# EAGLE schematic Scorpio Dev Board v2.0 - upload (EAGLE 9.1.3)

## Sheet 1 of 3: MAIN SECTION
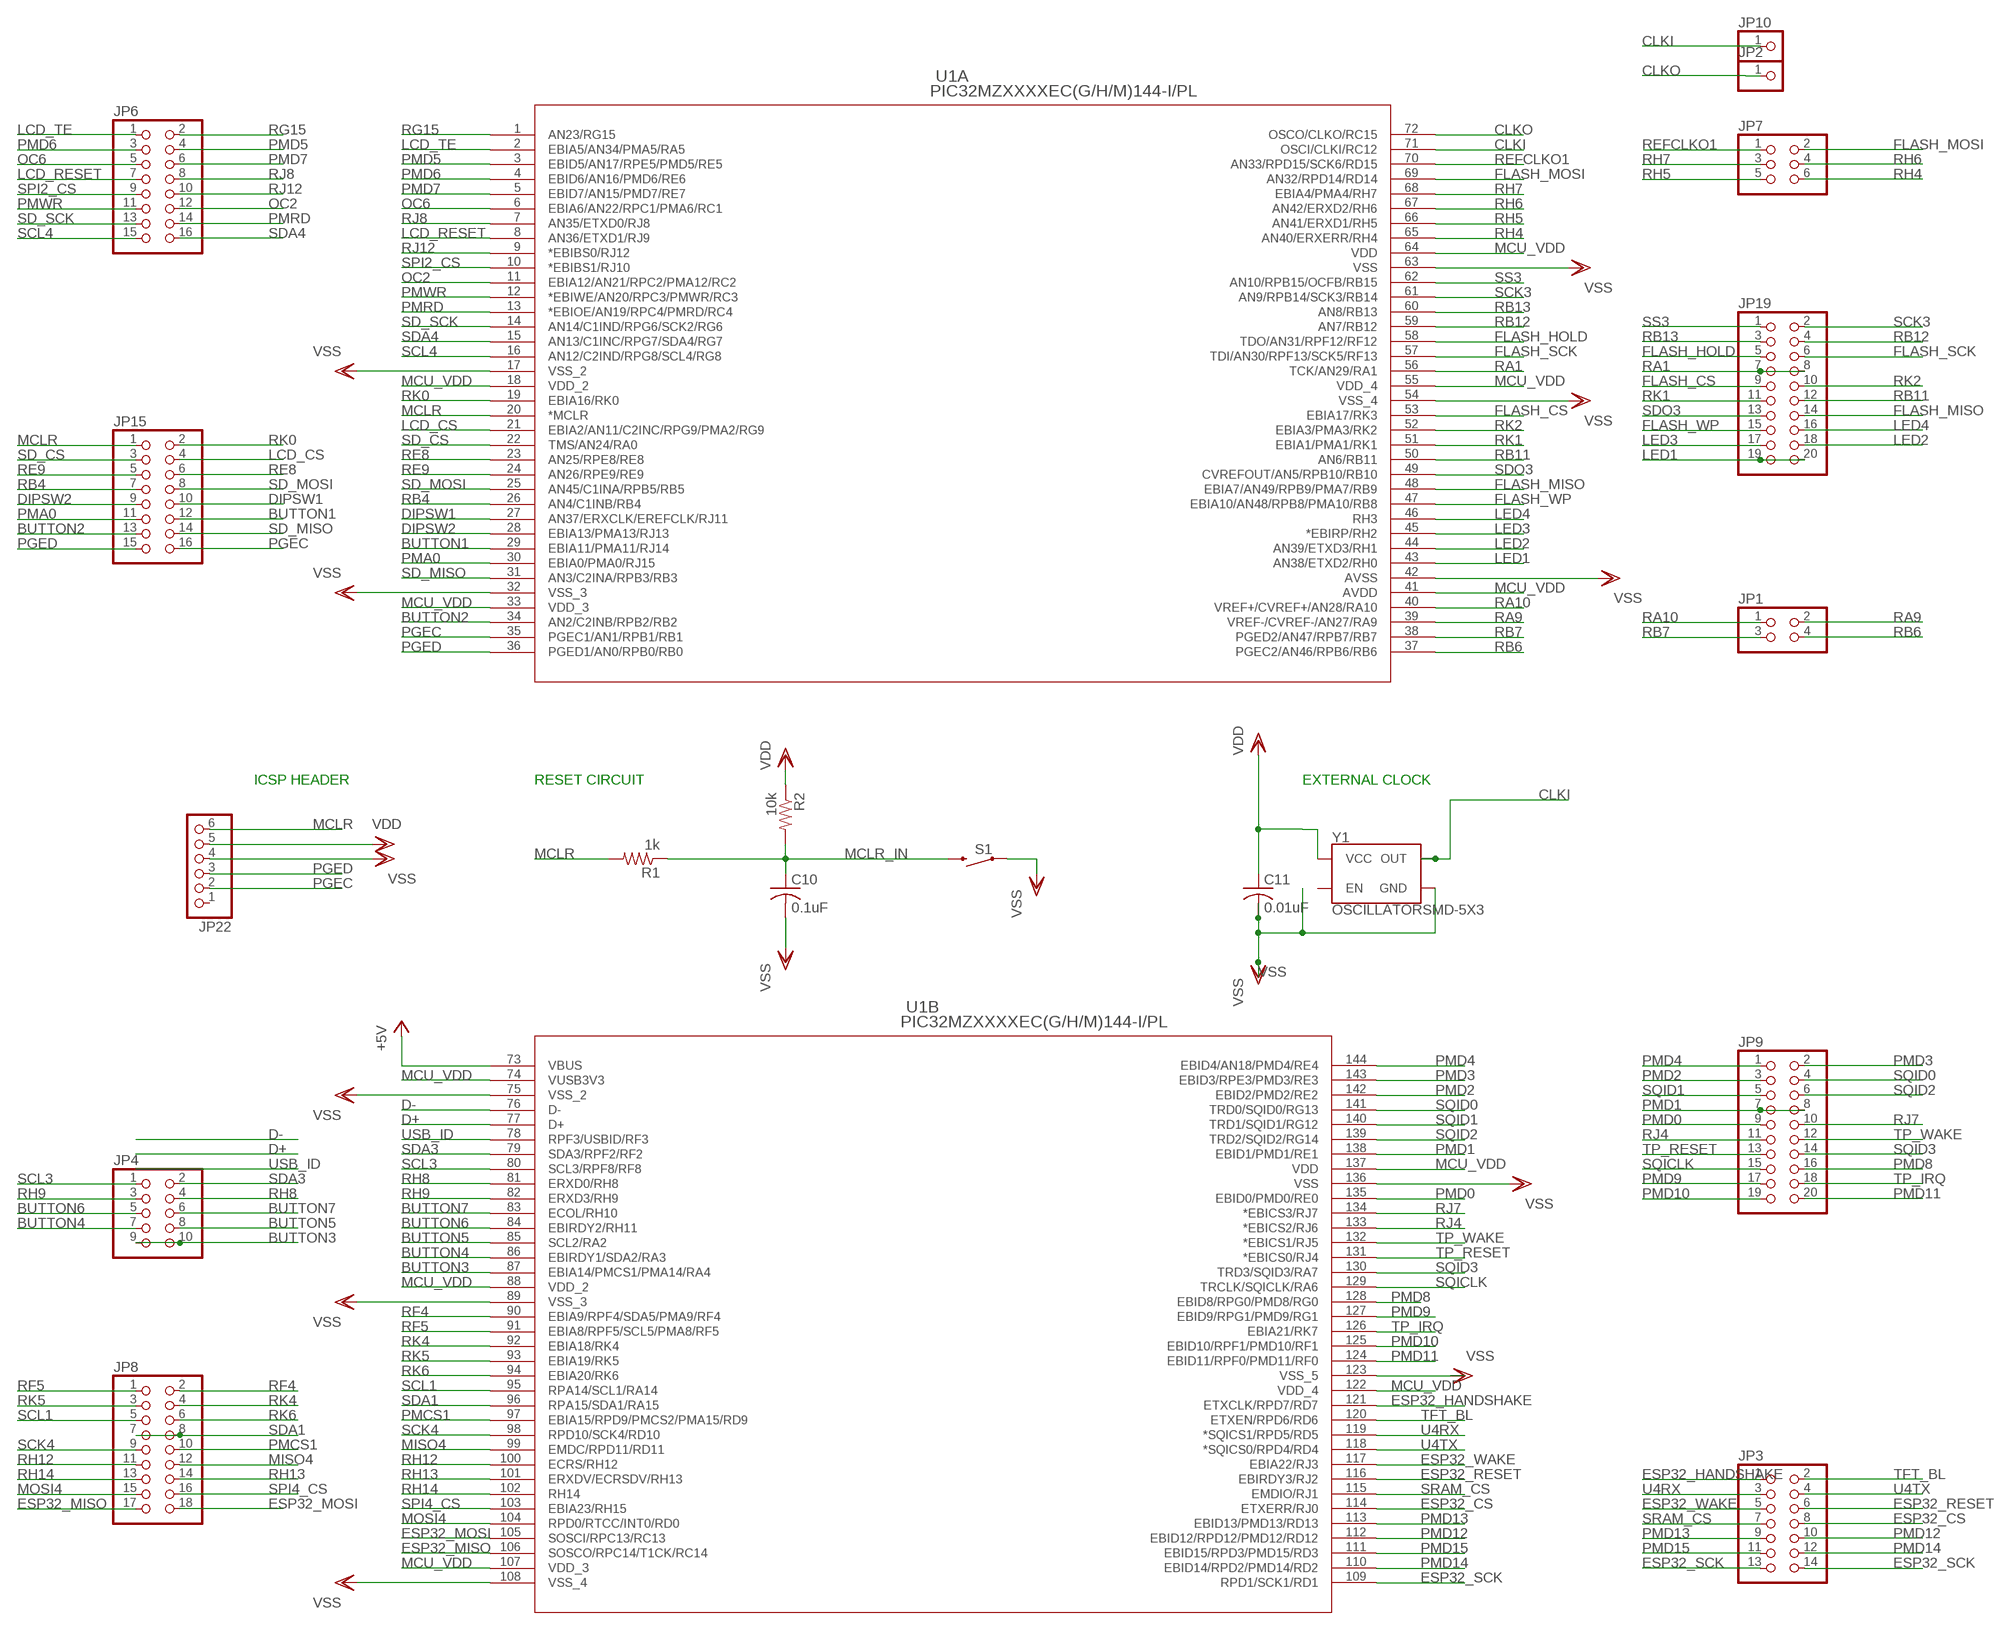
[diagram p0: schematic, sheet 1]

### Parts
C10  0.1uF  C-USC1206K  [C1206K]
C11  0.01uF  C-USC1206K  [C1206K]
JP1  PINHD-2X2  [2X02]
JP2  PINHD-1X1  [1X01]
JP3  PINHD-2X7  [2X07]
JP4  PINHD-2X5  [2X05]
JP6  PINHD-2X8  [2X08]
JP7  PINHD-2X3  [2X03]
JP8  PINHD-2X9  [2X09]
JP9  PINHD-2X10  [2X10]
JP10  PINHD-1X1  [1X01]
JP15  PINHD-2X8  [2X08]
JP19  PINHD-2X10  [2X10]
JP22  PINHD-1X6  [1X06]
R1  1k  R-US_M1206  [M1206]
R2  10k  R-US_M1206  [M1206]
S1  SWITCH-MOMENTARY-2PTH  [TACTILE-PTH]
U1  PIC32MZXXXXEC(G/H/M)144-I/PL  [LQFP144_20X20MC]
Y1  OSCILLATORSMD-5X3  [OSCILLATOR-SMD-5X3.2]

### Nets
+5V: U1.73(B:VBUS) ; also sheet 2,3
BUTTON1: JP15.12 U1.29(A:EBIA11/PMA11/RJ14) ; also sheet 2
BUTTON2: JP15.13 U1.34(A:AN2/C2INB/RPB2/RB2)
BUTTON3: JP4.9 JP4.10 U1.87(B:EBIA14/PMCS1/PMA14/RA4)
BUTTON4: JP4.7 U1.86(B:EBIRDY1/SDA2/RA3)
BUTTON5: JP4.8 U1.85(B:SCL2/RA2)
BUTTON6: JP4.5 U1.84(B:EBIRDY2/RH11)
BUTTON7: JP4.6 U1.83(B:ECOL/RH10)
CLKI: JP10.1 U1.71(A:OSCI/CLKI/RC12) Y1.3(OUT)
CLKO: JP2.1 U1.72(A:OSCO/CLKO/RC15)
D+: U1.77(B:D+) ; also sheet 2
D-: U1.76(B:D-) ; also sheet 2
DIPSW1: JP15.10 U1.27(A:AN37/ERXCLK/EREFCLK/RJ11)
DIPSW2: JP15.9 U1.28(A:EBIA13/PMA13/RJ13)
ESP32_CS: JP3.8 U1.114(B:ETXERR/RJ0) ; also sheet 2
ESP32_HANDSHAKE: JP3.1 U1.121(B:ETXCLK/RPD7/RD7) ; also sheet 2
ESP32_MISO: JP8.17 U1.106(B:SOSCO/RPC14/T1CK/RC14) ; also sheet 2
ESP32_MOSI: JP8.18 U1.105(B:SOSCI/RPC13/RC13) ; also sheet 2
ESP32_RESET: JP3.6 U1.116(B:EBIRDY3/RJ2) ; also sheet 2
ESP32_SCK: JP3.13 JP3.14 U1.109(B:RPD1/SCK1/RD1) ; also sheet 2
ESP32_WAKE: JP3.5 U1.117(B:EBIA22/RJ3) ; also sheet 2
FLASH_CS: JP19.9 U1.53(A:EBIA17/RK3) ; also sheet 2
FLASH_HOLD: JP19.5 U1.58(A:TDO/AN31/RPF12/RF12)
FLASH_MISO: JP19.14 U1.48(A:EBIA7/AN49/RPB9/PMA7/RB9) ; also sheet 2
FLASH_MOSI: JP7.2 U1.69(A:AN32/RPD14/RD14) ; also sheet 2
FLASH_SCK: JP19.6 U1.57(A:TDI/AN30/RPF13/SCK5/RF13) ; also sheet 2
FLASH_WP: JP19.15 U1.47(A:EBIA10/AN48/RPB8/PMA10/RB8) ; also sheet 2
LCD_CS: JP15.4 U1.21(A:EBIA2/AN11/C2INC/RPG9/PMA2/RG9) ; also sheet 2
LCD_RESET: JP6.7 U1.8(A:AN36/ETXD1/RJ9) ; also sheet 2
LCD_TE: JP6.1 U1.2(A:EBIA5/AN34/PMA5/RA5) ; also sheet 2
LED1: JP19.19 JP19.20 U1.43(A:AN38/ETXD2/RH0) ; also sheet 2
LED2: JP19.18 U1.44(A:AN39/ETXD3/RH1) ; also sheet 2
LED3: JP19.17 U1.45(A:*EBIRP/RH2) ; also sheet 2
LED4: JP19.16 U1.46(A:RH3) ; also sheet 2
MCLR: JP15.1 JP22.6 R1.2 U1.20(A:*MCLR)
MCLR_IN: C10.1 R1.1 R2.2 S1.3
MCU_VDD: U1.18(A:VDD_2) U1.33(A:VDD_3) U1.41(A:AVDD) U1.55(A:VDD_4) U1.64(A:VDD) U1.74(B:VUSB3V3) U1.88(B:VDD_2) U1.107(B:VDD_3) U1.122(B:VDD_4) U1.137(B:VDD) ; also sheet 2,3
MISO4: JP8.12 U1.99(B:EMDC/RPD11/RD11)
MOSI4: JP8.15 U1.104(B:RPD0/RTCC/INT0/RD0)
OC2: JP6.12 U1.11(A:EBIA12/AN21/RPC2/PMA12/RC2) ; also sheet 2
OC6: JP6.5 U1.6(A:EBIA6/AN22/RPC1/PMA6/RC1) ; also sheet 2
PGEC: JP15.16 JP22.2 U1.35(A:PGEC1/AN1/RPB1/RB1)
PGED: JP15.15 JP22.3 U1.36(A:PGED1/AN0/RPB0/RB0)
PMA0: JP15.11 U1.30(A:EBIA0/PMA0/RJ15) ; also sheet 2
PMCS1: JP8.10 U1.97(B:EBIA15/RPD9/PMCS2/PMA15/RD9)
PMD0: JP9.9 U1.135(B:EBID0/PMD0/RE0) ; also sheet 2
PMD1: JP9.7 JP9.8 U1.138(B:EBID1/PMD1/RE1) ; also sheet 2
PMD2: JP9.3 U1.142(B:EBID2/PMD2/RE2) ; also sheet 2
PMD3: JP9.2 U1.143(B:EBID3/RPE3/PMD3/RE3) ; also sheet 2
PMD4: JP9.1 U1.144(B:EBID4/AN18/PMD4/RE4) ; also sheet 2
PMD5: JP6.4 U1.3(A:EBID5/AN17/RPE5/PMD5/RE5) ; also sheet 2
PMD6: JP6.3 U1.4(A:EBID6/AN16/PMD6/RE6) ; also sheet 2
PMD7: JP6.6 U1.5(A:EBID7/AN15/PMD7/RE7) ; also sheet 2
PMD8: JP9.16 U1.128(B:EBID8/RPG0/PMD8/RG0) ; also sheet 2
PMD9: JP9.17 U1.127(B:EBID9/RPG1/PMD9/RG1) ; also sheet 2
PMD10: JP9.19 U1.125(B:EBID10/RPF1/PMD10/RF1) ; also sheet 2
PMD11: JP9.20 U1.124(B:EBID11/RPF0/PMD11/RF0) ; also sheet 2
PMD12: JP3.10 U1.112(B:EBID12/RPD12/PMD12/RD12) ; also sheet 2
PMD13: JP3.9 U1.113(B:EBID13/PMD13/RD13) ; also sheet 2
PMD14: JP3.12 U1.110(B:EBID14/RPD2/PMD14/RD2) ; also sheet 2
PMD15: JP3.11 U1.111(B:EBID15/RPD3/PMD15/RD3) ; also sheet 2
PMRD: JP6.14 U1.13(A:*EBIOE/AN19/RPC4/PMRD/RC4) ; also sheet 2
PMWR: JP6.11 U1.12(A:*EBIWE/AN20/RPC3/PMWR/RC3) ; also sheet 2
RA1: JP19.7 JP19.8 U1.56(A:TCK/AN29/RA1)
RA9: JP1.2 U1.39(A:VREF-/CVREF-/AN27/RA9)
RA10: JP1.1 U1.40(A:VREF+/CVREF+/AN28/RA10)
RB4: JP15.7 U1.26(A:AN4/C1INB/RB4)
RB6: JP1.4 U1.37(A:PGEC2/AN46/RPB6/RB6)
RB7: JP1.3 U1.38(A:PGED2/AN47/RPB7/RB7)
RB11: JP19.12 U1.50(A:AN6/RB11)
RB12: JP19.4 U1.59(A:AN7/RB12)
RB13: JP19.3 U1.60(A:AN8/RB13)
RE8: JP15.6 U1.23(A:AN25/RPE8/RE8)
RE9: JP15.5 U1.24(A:AN26/RPE9/RE9)
REFCLKO1: JP7.1 U1.70(A:AN33/RPD15/SCK6/RD15) ; also sheet 2
RF4: JP8.2 U1.90(B:EBIA9/RPF4/SDA5/PMA9/RF4)
RF5: JP8.1 U1.91(B:EBIA8/RPF5/SCL5/PMA8/RF5)
RG15: JP6.2 U1.1(A:AN23/RG15)
RH4: JP7.6 U1.65(A:AN40/ERXERR/RH4)
RH5: JP7.5 U1.66(A:AN41/ERXD1/RH5)
RH6: JP7.4 U1.67(A:AN42/ERXD2/RH6)
RH7: JP7.3 U1.68(A:EBIA4/PMA4/RH7)
RH8: JP4.4 U1.81(B:ERXD0/RH8)
RH9: JP4.3 U1.82(B:ERXD3/RH9)
RH12: JP8.11 U1.100(B:ECRS/RH12)
RH13: JP8.14 U1.101(B:ERXDV/ECRSDV/RH13)
RH14: JP8.13 U1.102(B:RH14)
RJ4: JP9.11 U1.133(B:*EBICS2/RJ6)
RJ7: JP9.10 U1.134(B:*EBICS3/RJ7)
RJ8: JP6.8 U1.7(A:AN35/ETXD0/RJ8)
RJ12: JP6.10 U1.9(A:*EBIBS0/RJ12)
RK0: JP15.2 U1.19(A:EBIA16/RK0)
RK1: JP19.11 U1.51(A:EBIA1/PMA1/RK1)
RK2: JP19.10 U1.52(A:EBIA3/PMA3/RK2)
RK4: JP8.4 U1.92(B:EBIA18/RK4)
RK5: JP8.3 U1.93(B:EBIA19/RK5)
RK6: JP8.6 U1.94(B:EBIA20/RK6)
SCK3: JP19.2 U1.61(A:AN9/RPB14/SCK3/RB14) ; also sheet 2
SCK4: JP8.9 U1.98(B:RPD10/SCK4/RD10)
SCL1: JP8.5 U1.95(B:RPA14/SCL1/RA14) ; also sheet 2
SCL3: JP4.1 U1.80(B:SCL3/RPF8/RF8)
SCL4: JP6.15 U1.16(A:AN12/C2IND/RPG8/SCL4/RG8) ; also sheet 2
SD_CS: JP15.3 U1.22(A:TMS/AN24/RA0) ; also sheet 2
SD_MISO: JP15.14 U1.31(A:AN3/C2INA/RPB3/RB3) ; also sheet 2
SD_MOSI: JP15.8 U1.25(A:AN45/C1INA/RPB5/RB5) ; also sheet 2
SD_SCK: JP6.13 U1.14(A:AN14/C1IND/RPG6/SCK2/RG6) ; also sheet 2
SDA1: JP8.7 JP8.8 U1.96(B:RPA15/SDA1/RA15) ; also sheet 2
SDA3: JP4.2 U1.79(B:SDA3/RPF2/RF2)
SDA4: JP6.16 U1.15(A:AN13/C1INC/RPG7/SDA4/RG7) ; also sheet 2
SDO3: JP19.13 U1.49(A:CVREFOUT/AN5/RPB10/RB10) ; also sheet 2
SPI2_CS: JP6.9 U1.10(A:*EBIBS1/RJ10)
SPI4_CS: JP8.16 U1.103(B:EBIA23/RH15)
SQICLK: JP9.15 U1.129(B:TRCLK/SQICLK/RA6) ; also sheet 2
SQID0: JP9.4 U1.141(B:TRD0/SQID0/RG13) ; also sheet 2
SQID1: JP9.5 U1.140(B:TRD1/SQID1/RG12) ; also sheet 2
SQID2: JP9.6 U1.139(B:TRD2/SQID2/RG14) ; also sheet 2
SQID3: JP9.14 U1.130(B:TRD3/SQID3/RA7) ; also sheet 2
SRAM_CS: JP3.7 U1.115(B:EMDIO/RJ1) ; also sheet 2
SS3: JP19.1 U1.62(A:AN10/RPB15/OCFB/RB15) ; also sheet 2
TFT_BL: JP3.2 U1.120(B:ETXEN/RPD6/RD6) ; also sheet 2
TP_IRQ: JP9.18 U1.126(B:EBIA21/RK7) ; also sheet 2
TP_RESET: JP9.13 U1.131(B:*EBICS0/RJ4) ; also sheet 2
TP_WAKE: JP9.12 U1.132(B:*EBICS1/RJ5) ; also sheet 2
U4RX: JP3.3 U1.119(B:*SQICS1/RPD5/RD5) ; also sheet 2
U4TX: JP3.4 U1.118(B:*SQICS0/RPD4/RD4) ; also sheet 2
USB_ID: U1.78(B:RPF3/USBID/RF3) ; also sheet 2
VDD: C11.1 JP22.5 R2.1 Y1.4(VCC) ; also sheet 2,3
VSS: C10.2 C11.2 JP22.4 S1.1 U1.17(A:VSS_2) U1.32(A:VSS_3) U1.42(A:AVSS) U1.54(A:VSS_4) U1.63(A:VSS) U1.75(B:VSS_2) U1.89(B:VSS_3) U1.108(B:VSS_4) U1.123(B:VSS_5) U1.136(B:VSS) Y1.2(GND) ; also sheet 2,3
Unconnected: JP22.1 Y1.1(EN)

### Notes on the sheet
- ICSP HEADER | RESET CIRCUIT | EXTERNAL CLOCK

## Sheet 2 of 3: PERIPHERALS SECTION
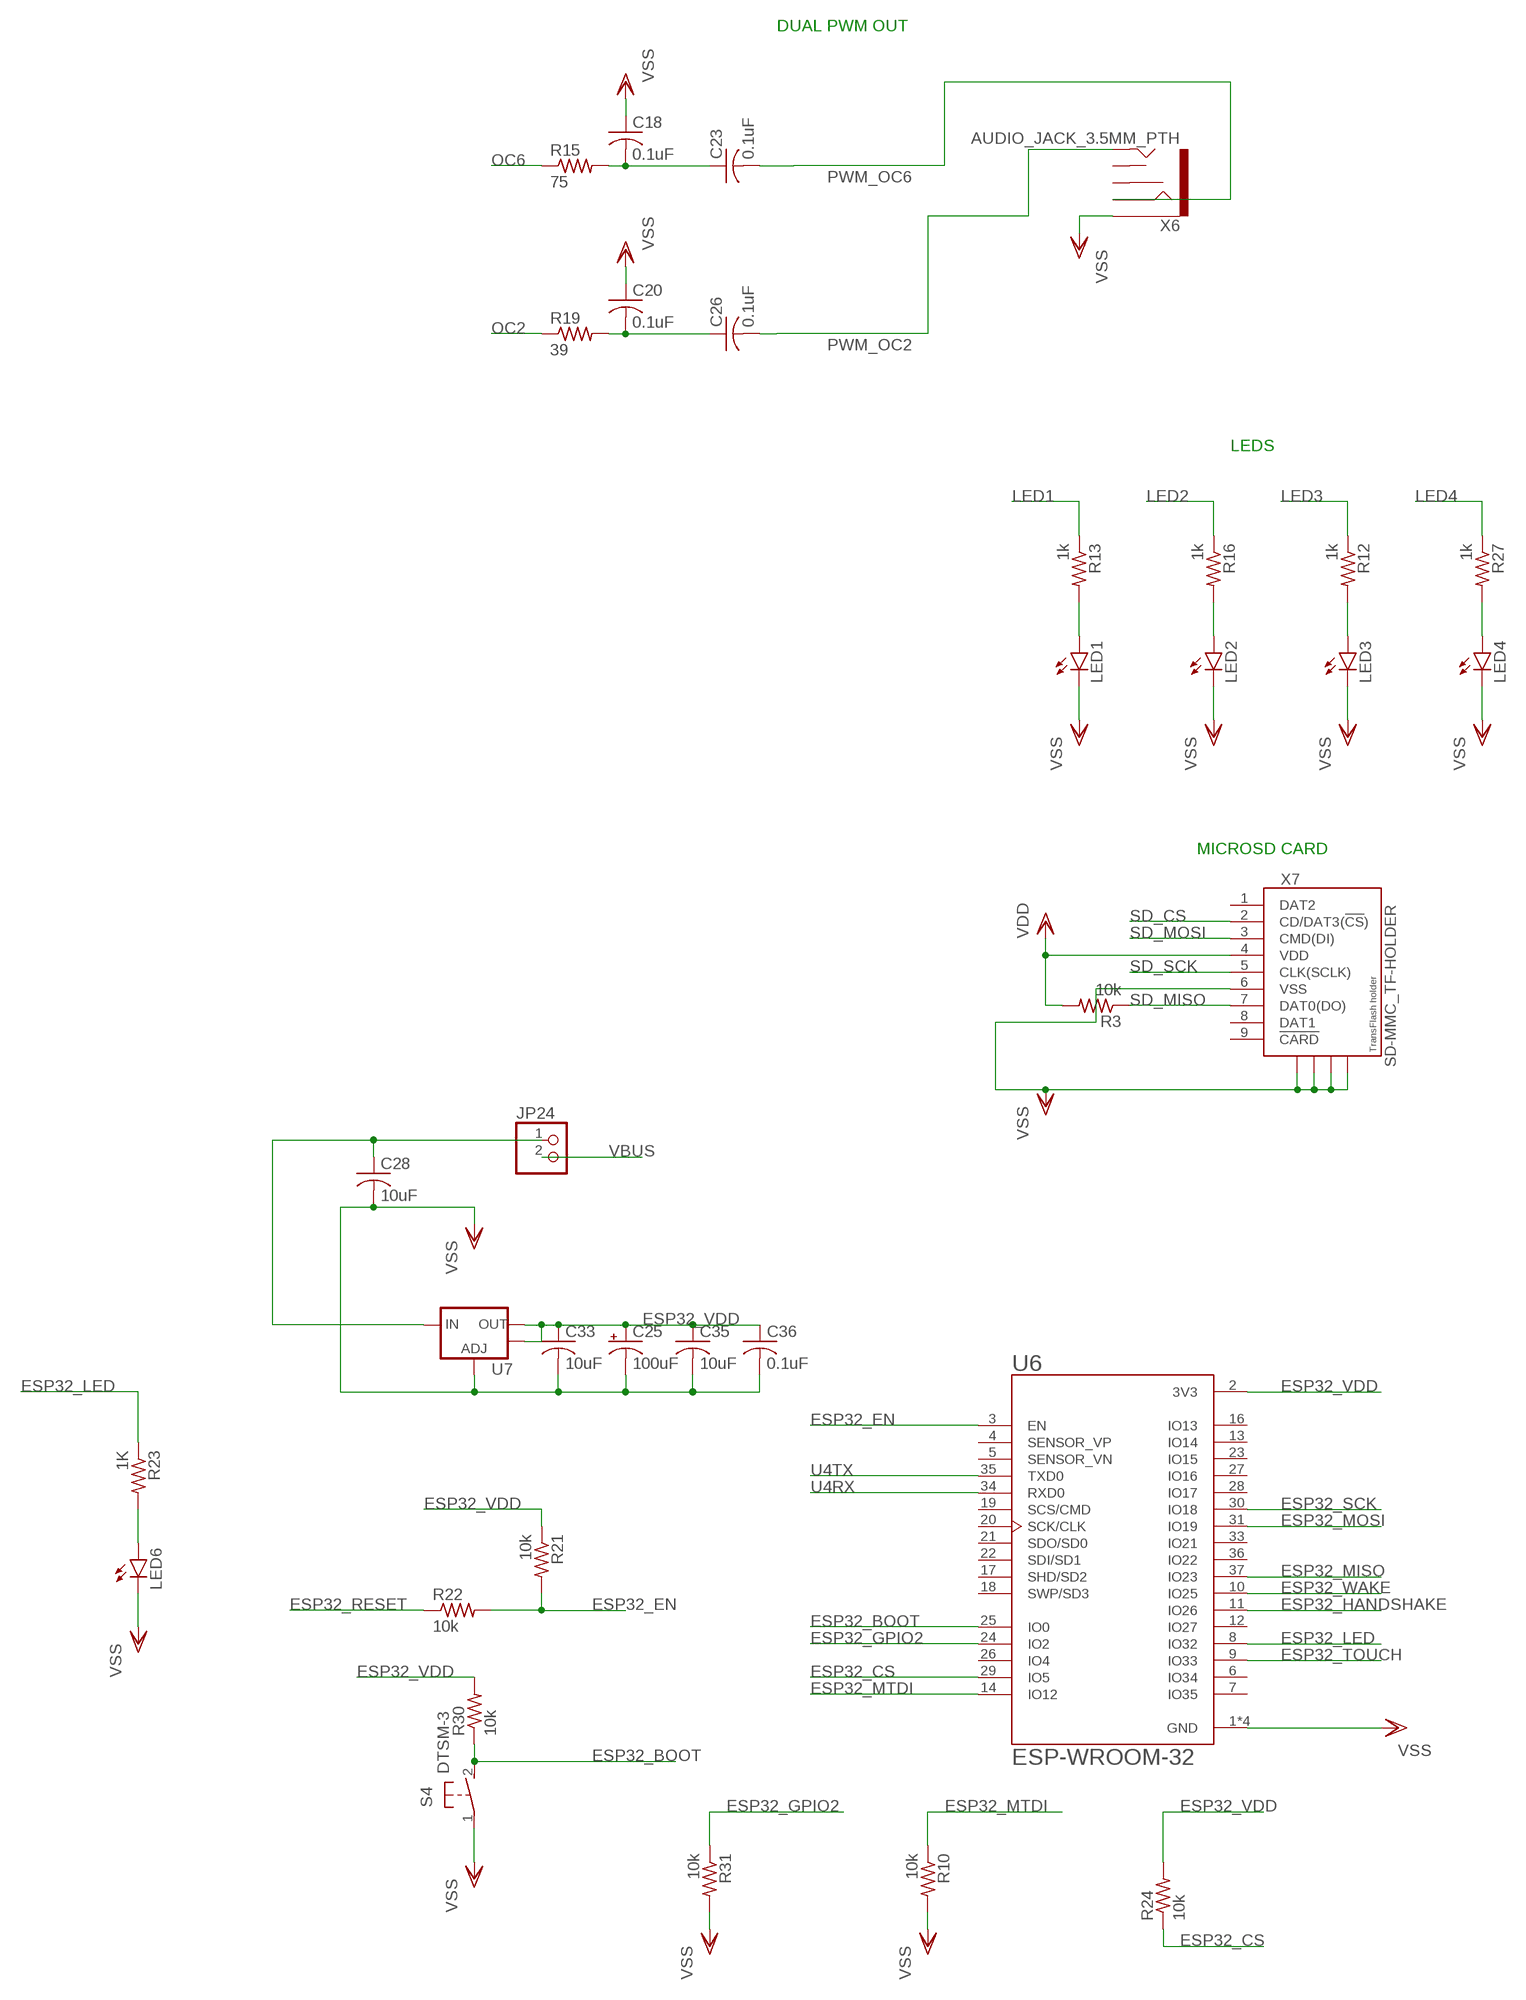
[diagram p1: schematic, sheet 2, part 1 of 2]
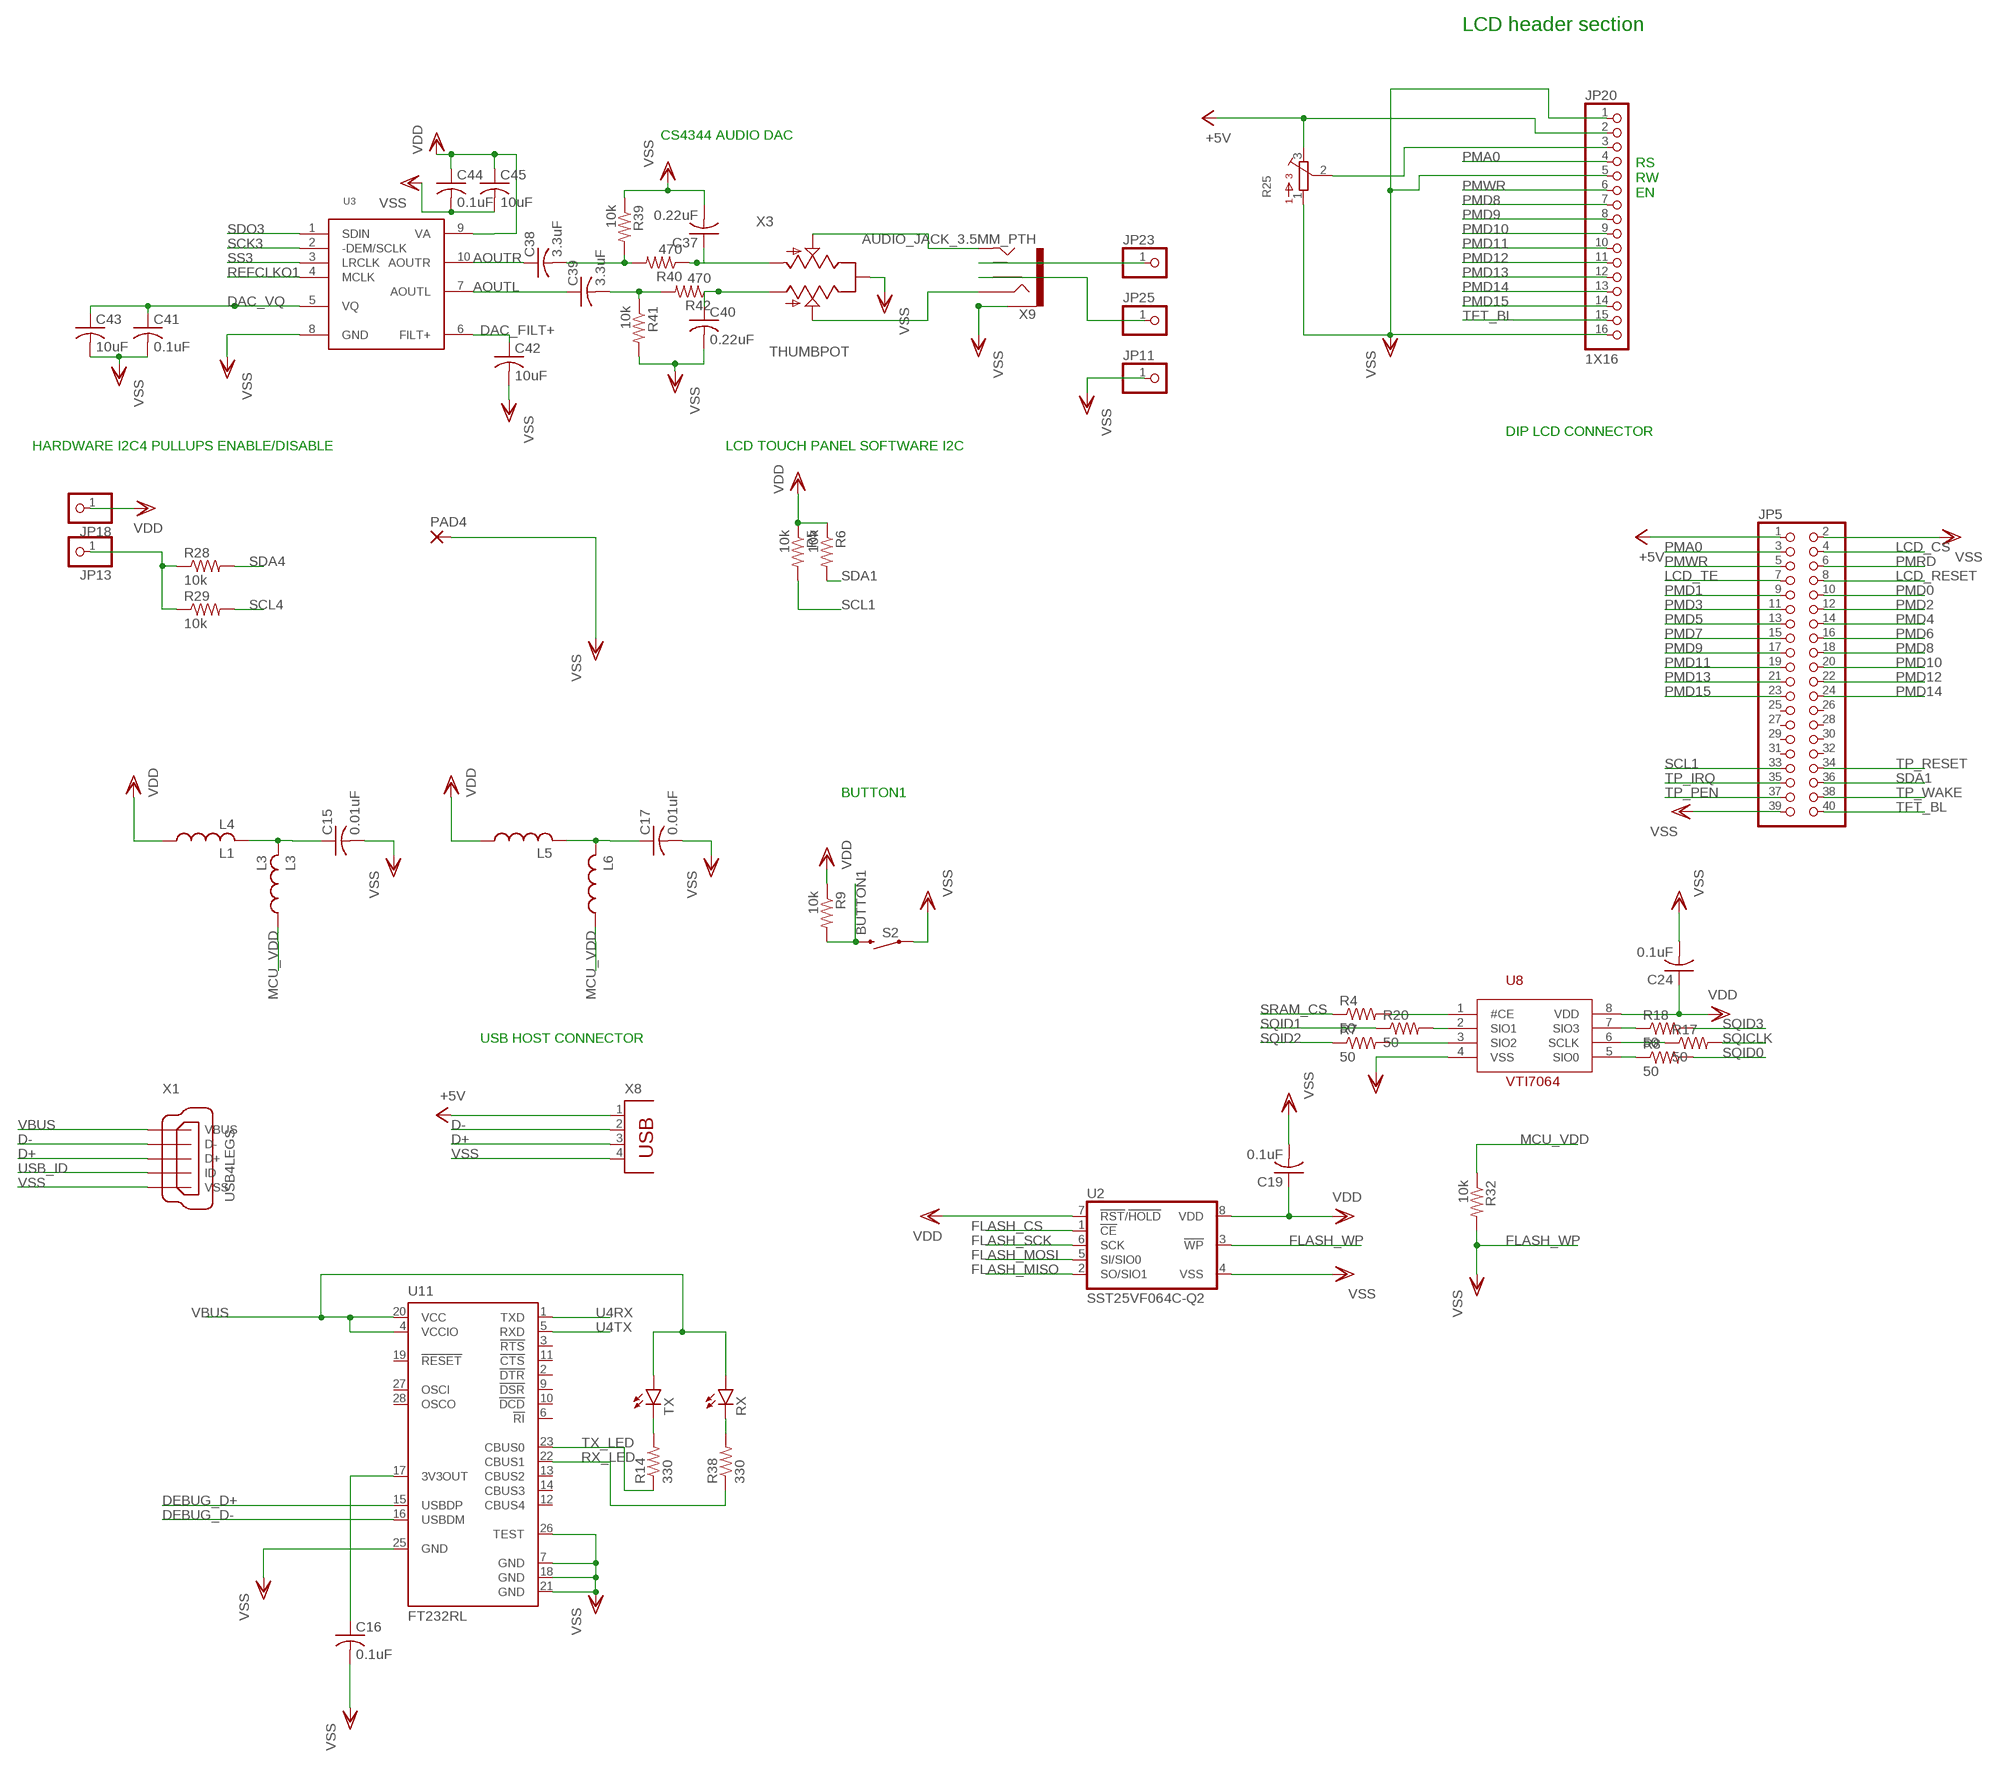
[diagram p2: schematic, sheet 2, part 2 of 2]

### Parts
C15  0.01uF  C-USC1206K  [C1206K]
C16  0.1uF  C-USC1206K  [C1206K]
C17  0.01uF  C-USC1206K  [C1206K]
C18  0.1uF  C-USC1206K  [C1206K]
C19  0.1uF  C-USC1206K  [C1206K]
C20  0.1uF  C-USC1206K  [C1206K]
C23  0.1uF  C-USC1206K  [C1206K]
C24  0.1uF  C-USC1206K  [C1206K]
C25  100uF  CPOL-USB/3528-21W  [B/3528-21W]
C26  0.1uF  C-USC1206K  [C1206K]
C28  10uF  C-USC1206K  [C1206K]
C33  10uF  C-USC1206K  [C1206K]
C35  10uF  C-USC1206K  [C1206K]
C36  0.1uF  C-USC1206K  [C1206K]
C37  0.22uF  C-USC1206K  [C1206K]
C38  3.3uF  C-USC1206K  [C1206K]
C39  3.3uF  C-USC1206K  [C1206K]
C40  0.22uF  C-USC1206K  [C1206K]
C41  0.1uF  C-USC1206K  [C1206K]
C42  10uF  C-USC1206K  [C1206K]
C43  10uF  C-USC1206K  [C1206K]
C44  0.1uF  C-USC1206K  [C1206K]
C45  10uF  C-USC1206K  [C1206K]
JP5  PINHD-2X20  [2X20]
JP11  PINHD-1X1  [1X01]
JP13  PINHD-1X1  [1X01]
JP18  PINHD-1X1  [1X01]
JP20  1X16  [1X16]
JP23  PINHD-1X1  [1X01]
JP24  PINHD-1X2  [1X02]
JP25  PINHD-1X1  [1X01]
L1  L4  L-USL3216C  [L3216C]
L3  L3  L-USL3216C  [L3216C]
L5  L-USL3216C  [L3216C]
L6  L-USL3216C  [L3216C]
LED1  LEDSMT1206  [1206]
LED2  LEDSMT1206  [1206]
LED3  LEDSMT1206  [1206]
LED4  LEDSMT1206  [1206]
LED6  LEDSMT1206  [1206]
PAD4  SMD5  [SMD2,54-5,08]
R3  10k  R-US_M1206  [M1206]
R4  50  R-US_M1206  [M1206]
R5  10k  R-US_M1206  [M1206]
R6  10k  R-US_M1206  [M1206]
R7  50  R-US_M1206  [M1206]
R8  50  R-US_M1206  [M1206]
R9  10k  R-US_M1206  [M1206]
R10  10k  R-US_M1206  [M1206]
R12  1k  R-US_M1206  [M1206]
R13  1k  R-US_M1206  [M1206]
R14  330  R-US_R0603  [R0603]
R15  75  R-US_R1206  [R1206]
R16  1k  R-US_M1206  [M1206]
R17  50  R-US_M1206  [M1206]
R18  50  R-US_M1206  [M1206]
R19  39  R-US_R1206  [R1206]
R20  50  R-US_M1206  [M1206]
R21  10k  R-US_M1206  [M1206]
R22  10k  R-US_M1206  [M1206]
R23  1K  R-US_M1206  [M1206]
R24  10k  R-US_M1206  [M1206]
R25  3386-X  [3386X]
R27  1k  R-US_M1206  [M1206]
R28  10k  R-US_M1206  [M1206]
R29  10k  R-US_M1206  [M1206]
R30  10k  R-US_M1206  [M1206]
R31  10k  R-US_M1206  [M1206]
R32  10k  R-US_M1206  [M1206]
R38  330  R-US_R0603  [R0603]
R39  10k  R-US_M1206  [M1206]
R40  470  R-US_M1206  [M1206]
R41  10k  R-US_M1206  [M1206]
R42  470  R-US_M1206  [M1206]
RX  LEDSMT1206  [1206]
S2  SWITCH-MOMENTARY-2PTH  [TACTILE-PTH]
S4  DTSM-3  [DTSM-3]
TX  LEDSMT1206  [1206]
U2  SST25VF064C-Q2  [WSON8-Q2A]
U3  CS4344  [MSOP10]
U6  ESP-WROOM-32  [MODULE_ESP-WROOM-32]
U7  V_REG_LM1117SOT223  [SOT223]
U8  VTI7064  [SOIC8]
U11  FT232RL  [SSOP28]
X1  USB4LEGS  LCSC_MICRO_USB_4_LEGS  [LCSC_MICRO_USB_4_LEGS]
X3  THUMBPOT  [TRIM_A14061600UX0005]
X6  AUDIO_JACK_3.5MM_PTH  [AUDIO-JACK]
X7  SD-MMC_TF-HOLDER  [SD-MMC_TF-PULL]
X8  PN87520  [PN87520]
X9  AUDIO_JACK_3.5MM_PTH  [AUDIO-JACK]

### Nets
+5V: JP5.1 JP20.2 R25.3 X8.1 ; also sheet 1,3
AOUTL: C39.1 U3.7(AOUTL)
AOUTR: C38.1 U3.10(AOUTR)
BUTTON1: R9.2 S2.3 ; also sheet 1
D+: X1.D+ X8.3 ; also sheet 1
D-: X1.D- X8.2 ; also sheet 1
DAC_FILT+: C42.1 U3.6(FILT+)
DAC_VQ: C41.1 C43.1 U3.5(VQ)
DEBUG_D+: U11.15(USBDP) ; also sheet 3
DEBUG_D-: U11.16(USBDM) ; also sheet 3
ESP32_BOOT: R30.1 S4.2 U6.25(IO0)
ESP32_CS: R24.1 U6.29(IO5) ; also sheet 1
ESP32_EN: R21.2 R22.2 U6.3(EN)
ESP32_GPIO2: R31.1 U6.24(IO2)
ESP32_HANDSHAKE: U6.11(IO26) ; also sheet 1
ESP32_LED: R23.1 U6.8(IO32)
ESP32_MISO: U6.37(IO23) ; also sheet 1
ESP32_MOSI: U6.31(IO19) ; also sheet 1
ESP32_MTDI: R10.1 U6.14(IO12)
ESP32_RESET: R22.1 ; also sheet 1
ESP32_SCK: U6.30(IO18) ; also sheet 1
ESP32_TOUCH: U6.9(IO33)
ESP32_VDD: C25.+ C33.1 C35.1 C36.1 R21.1 R24.2 R30.2 U6.2(3V3) U7.2(OUT) U7.4(OUT)
ESP32_WAKE: U6.10(IO25) ; also sheet 1
FLASH_CS: U2.1(!CE!) ; also sheet 1
FLASH_MISO: U2.2(SO/SIO1) ; also sheet 1
FLASH_MOSI: U2.5(SI/SIO0) ; also sheet 1
FLASH_SCK: U2.6(SCK) ; also sheet 1
FLASH_WP: R32.2 U2.3(!WP!) ; supply symbol labelled VSS ; also sheet 1
LCD_CS: JP5.4 ; also sheet 1
LCD_RESET: JP5.8 ; also sheet 1
LCD_TE: JP5.7 ; also sheet 1
LED1: R13.1 ; also sheet 1
LED2: R16.1 ; also sheet 1
LED3: R12.1 ; also sheet 1
LED4: R27.1 ; also sheet 1
MCU_VDD: L3.1 L6.1 R32.1 ; also sheet 1,3
N$1: JP20.3 R25.2
N$2: LED3.A R12.2
N$3: LED6.A R23.2
N$6: C20.2 C26.1 R19.2
N$7: LED4.A R27.2
N$8: JP13.1 R28.1 R29.1
N$11: R20.2 U8.2(SIO1)
N$12: JP23.1 X9.TSH
N$14: R4.2 U8.1(#CE)
N$15: R7.2 U8.3(SIO2)
N$19: R8.1 U8.5(SIO0)
N$20: JP25.1 X9.RSH
N$21: R17.1 U8.6(SCLK)
N$22: X3.3(3/OUT2) X9.TIP
N$23: X3.2(2/OUT1) X9.RING
N$24: C16.1 U11.17(3V3OUT)
N$25: C28.1 JP24.1 U7.3(IN)
N$26: C18.2 C23.1 R15.2
N$27: LED1.A R13.2
N$31: R18.1 U8.7(SIO3)
N$32: C15.1 L1.2 L3.2
N$33: C17.1 L5.2 L6.2
N$34: C40.1 R42.1 X3.4(4/IN1)
N$35: C39.2 R41.1 R42.2
N$38: C38.2 R39.2 R40.2
N$39: C37.1 R40.1 X3.5(5/IN2)
N$46: R14.2 TX.C
N$63: R38.2 RX.C
N$80: LED2.A R16.2
OC2: R19.1 ; also sheet 1
OC6: R15.1 ; also sheet 1
PMA0: JP5.3 JP20.4 ; also sheet 1
PMD0: JP5.10 ; also sheet 1
PMD1: JP5.9 ; also sheet 1
PMD2: JP5.12 ; also sheet 1
PMD3: JP5.11 ; also sheet 1
PMD4: JP5.14 ; also sheet 1
PMD5: JP5.13 ; also sheet 1
PMD6: JP5.16 ; also sheet 1
PMD7: JP5.15 ; also sheet 1
PMD8: JP5.18 JP20.7 ; also sheet 1
PMD9: JP5.17 JP20.8 ; also sheet 1
PMD10: JP5.20 JP20.9 ; also sheet 1
PMD11: JP5.19 JP20.10 ; also sheet 1
PMD12: JP5.22 JP20.11 ; also sheet 1
PMD13: JP5.21 JP20.12 ; also sheet 1
PMD14: JP5.24 JP20.13 ; also sheet 1
PMD15: JP5.23 JP20.14 ; also sheet 1
PMRD: JP5.6 ; also sheet 1
PMWR: JP5.5 JP20.6 ; also sheet 1
PWM_OC2: C26.2 X6.TIP
PWM_OC6: C23.2 X6.RING
REFCLKO1: U3.4(MCLK) ; also sheet 1
RX_LED: R38.1 U11.22(CBUS1)
SCK3: U3.2(-DEM/SCLK) ; also sheet 1
SCL1: JP5.33 R5.2 ; also sheet 1
SCL4: R29.2 ; also sheet 1
SD_CS: X7.2(CD/DAT3(!CS!)) ; also sheet 1
SD_MISO: R3.1 X7.7(DAT0(DO)) ; also sheet 1
SD_MOSI: X7.3(CMD(DI)) ; also sheet 1
SD_SCK: X7.5(CLK(SCLK)) ; also sheet 1
SDA1: JP5.36 R6.2 ; also sheet 1
SDA4: R28.2 ; also sheet 1
SDO3: U3.1(SDIN) ; also sheet 1
SQICLK: R17.2 ; also sheet 1
SQID0: R8.2 ; also sheet 1
SQID1: R20.1 ; also sheet 1
SQID2: R7.1 ; also sheet 1
SQID3: R18.2 ; also sheet 1
SRAM_CS: R4.1 ; also sheet 1
SS3: U3.3(LRCLK) ; also sheet 1
TFT_BL: JP5.40 JP20.15 ; also sheet 1
TP_IRQ: JP5.35 ; also sheet 1
TP_PEN: JP5.37
TP_RESET: JP5.34 ; also sheet 1
TP_WAKE: JP5.38 ; also sheet 1
TX_LED: R14.1 U11.23(CBUS0)
U4RX: U6.34(RXD0) U11.1(TXD) ; also sheet 1
U4TX: U6.35(TXD0) U11.5(RXD) ; also sheet 1
USB_ID: X1.ID ; also sheet 1
VBUS: JP24.2 RX.A TX.A U11.4(VCCIO) U11.20(VCC) X1.VBUS ; also sheet 3
VDD: C19.1 C24.1 C44.1 C45.1 JP18.1 L1.1 L5.1 R3.2 R5.1 R6.1 R9.1 U2.7(!RST!/!HOLD!) U2.8(VDD) U3.9(VA) U8.8(VDD) X7.4(VDD) ; also sheet 1,3
VSS: C15.2 C16.2 C17.2 C18.1 C19.2 C20.1 C24.2 C25.- C28.2 C33.2 C35.2 C36.2 C37.2 C40.2 C41.2 C42.2 C43.2 C44.2 C45.2 JP5.2 JP5.39 JP11.1 JP20.1 JP20.5 JP20.16 LED1.C LED2.C LED3.C LED4.C LED6.C PAD4.1(P) R10.2 R25.1 R31.2 R39.1 R41.2 S2.1 S4.1 U2.4(VSS) U3.8(GND) U6.1(GND) U6.1.1(GND) U6.15(GND) U6.38(GND) U7.1(ADJ) U8.4(VSS) U11.7(GND) U11.18(GND) U11.21(GND) U11.25(GND) U11.26(TEST) X1.GND(VSS) X3.1(1/COMMON) X6.SLEEVE X7.6(VSS) X7.S1 X7.S2 X7.S3 X7.S4 X8.4 X9.SLEEVE ; also sheet 1,3
Unconnected: JP5.25 JP5.26 JP5.27 JP5.28 JP5.29 JP5.30 JP5.31 JP5.32 U6.4(SENSOR_VP) U6.5(SENSOR_VN) U6.6(IO34) U6.7(IO35) U6.12(IO27) U6.13(IO14) U6.16(IO13) U6.17(SHD/SD2) U6.18(SWP/SD3) U6.19(SCS/CMD) U6.20(SCK/CLK) U6.21(SDO/SD0) U6.22(SDI/SD1) U6.23(IO15) U6.26(IO4) U6.27(IO16) U6.28(IO17) U6.33(IO21) U6.36(IO22) U11.2(!DTR) U11.3(!RTS) U11.6(!RI) U11.9(!DSR) U11.10(!DCD) U11.11(!CTS) U11.12(CBUS4) U11.13(CBUS2) U11.14(CBUS3) U11.19(!RESET) U11.27(OSCI) U11.28(OSCO) X6.RSH X6.TSH X7.1(DAT2) X7.8(DAT1) X7.9(!CARD)

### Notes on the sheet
- LCD header section
- DUAL PWM OUT
- CS4344 AUDIO DAC
- RS
  RW
  EN
- DIP LCD CONNECTOR
- LEDS | HARDWARE I2C4 PULLUPS ENABLE/DISABLE | LCD TOUCH PANEL SOFTWARE I2C
- MICROSD CARD | BUTTON1
- USB HOST CONNECTOR

## Sheet 3 of 3: POWER SECTION
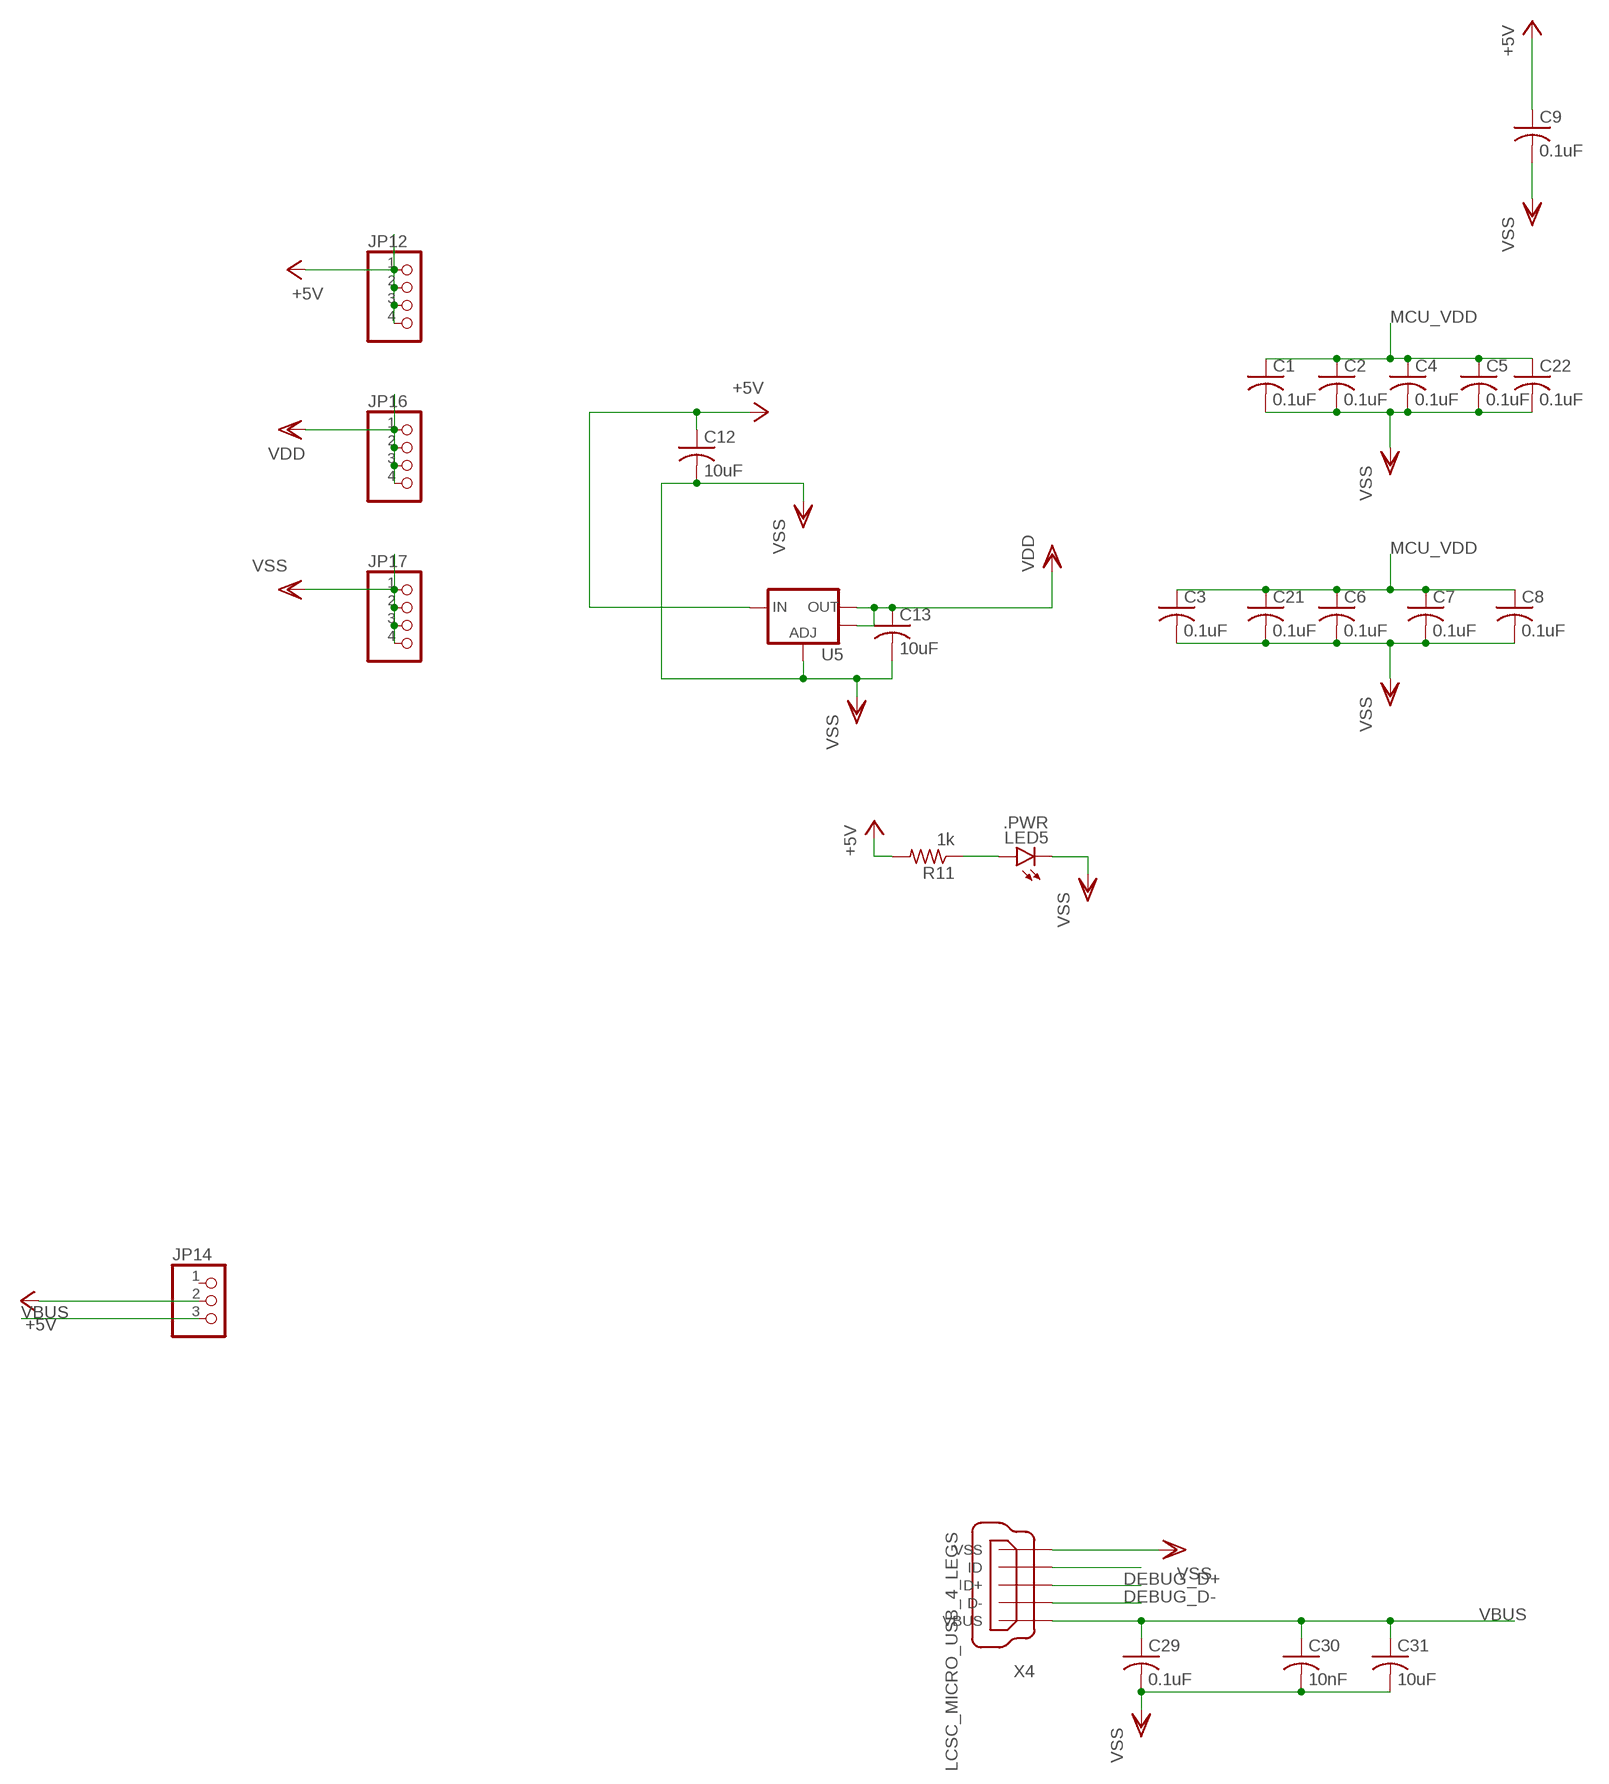
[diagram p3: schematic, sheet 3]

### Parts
C1  0.1uF  C-USC1206K  [C1206K]
C2  0.1uF  C-USC1206K  [C1206K]
C3  0.1uF  C-USC1206K  [C1206K]
C4  0.1uF  C-USC1206K  [C1206K]
C5  0.1uF  C-USC1206K  [C1206K]
C6  0.1uF  C-USC1206K  [C1206K]
C7  0.1uF  C-USC1206K  [C1206K]
C8  0.1uF  C-USC1206K  [C1206K]
C9  0.1uF  C-USC1206K  [C1206K]
C12  10uF  C-USC1206K  [C1206K]
C13  10uF  C-USC1206K  [C1206K]
C21  0.1uF  C-USC1206K  [C1206K]
C22  0.1uF  C-USC1206K  [C1206K]
C29  0.1uF  C-USC1206K  [C1206K]
C30  10nF  C-USC1206K  [C1206K]
C31  10uF  C-USC1206K  [C1206K]
JP12  PINHD-1X4  [1X04]
JP14  PINHD-1X3  [1X03]
JP16  PINHD-1X4  [1X04]
JP17  PINHD-1X4  [1X04]
LED5  .PWR  LEDSMT1206  [1206]
R11  1k  R-US_M1206  [M1206]
U5  V_REG_LM1117SOT223  [SOT223]
X4  LCSC_MICRO_USB_4_LEGS  [LCSC_MICRO_USB_4_LEGS]

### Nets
+5V: C9.1 C12.1 JP12.1 JP12.2 JP12.3 JP12.4 JP14.2 R11.2 U5.3(IN) ; also sheet 1,2
DEBUG_D+: X4.D+ ; also sheet 2
DEBUG_D-: X4.D- ; also sheet 2
MCU_VDD: C1.1 C2.1 C3.1 C4.1 C5.1 C6.1 C7.1 C8.1 C21.1 C22.1 ; also sheet 1,2
N$5: X4.ID
N$17: LED5.A R11.1
VBUS: C29.1 C30.1 C31.1 JP14.3 X4.VBUS ; also sheet 2
VDD: C13.1 JP16.1 JP16.2 JP16.3 JP16.4 U5.2(OUT) U5.4(OUT) ; also sheet 1,2
VSS: C1.2 C2.2 C3.2 C4.2 C5.2 C6.2 C7.2 C8.2 C9.2 C12.2 C13.2 C21.2 C22.2 C29.2 C30.2 C31.2 JP17.1 JP17.2 JP17.3 JP17.4 LED5.C U5.1(ADJ) X4.GND(VSS) ; also sheet 1,2
Unconnected: JP14.1

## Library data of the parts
C1-C13 C15-C24 C26 C28-C31 C33 C35-C45 = rcl:C-US: CAPACITOR, American symbol; SPICEPREFIX: C
C25 = rcl:CPOL-US: POLARIZED CAPACITOR, American symbol; SPICEPREFIX: C
JP1 = pinhead:PINHD-2X2: PIN HEADER
JP2 JP10 JP11 JP13 JP18 JP23 JP25 = pinhead:PINHD-1X1: PIN HEADER
JP3 = pinhead:PINHD-2X7: PIN HEADER
JP4 = pinhead:PINHD-2X5: PIN HEADER
JP5 = pinhead:PINHD-2X20: PIN HEADER
JP6 JP15 = pinhead:PINHD-2X8: PIN HEADER
JP7 = pinhead:PINHD-2X3: PIN HEADER
JP8 = pinhead:PINHD-2X9: PIN HEADER
JP9 JP19 = pinhead:PINHD-2X10: PIN HEADER
JP12 JP16 JP17 = pinhead:PINHD-1X4: PIN HEADER
JP14 = pinhead:PINHD-1X3: PIN HEADER
JP20 = mypinheaders:1X16
JP22 = pinhead:PINHD-1X6: PIN HEADER
JP24 = pinhead:PINHD-1X2: PIN HEADER
L1 L3 L5 L6 = rcl:L-US: INDUCTOR, American symbol; SPICEPREFIX: L
LED1-LED6 RX TX = led:LED: LED
PAD4 = wirepad:SMD5: SMD PAD
R1-R24 R27-R32 R38-R42 = rcl:R-US_: RESISTOR, American symbol; SPICEPREFIX: R
R25 = bourns:3386-: 3386 Series 3/8" Square Trimmer
S1 S2 = test:SWITCH-MOMENTARY-2: Various NO switches- pushbuttons, reed, etc; PROD_ID: SWCH-08441
S4 = switch-tact:DTSM-3
U1 = PIC32MZ:PIC32MZXXXXEC(G/H/M)144-I/PL; MANUFACTURER_PART_NUMBER: pic32mz2048ech144-i/pl; VENDOR: Microchip
U2 = memory-sst:SST25VF064C: EEPROM 64 Mbit SPI Serial Dual I/O Flash
U3 = cirrus-3:CS4344
U5 U7 = SparkFun:V_REG_LM1117: Voltage Regulator LM1117 Standard adjustable voltage regulator but in SMD form. Spark Fun Electronics SKU : COM-00595
U6 = ESP-WROOM-32:ESP-WROOM-32: Module: combo; GPIO, I2C x2, I2S x2, SDIO, SPI x3, UART x3; 19.5dBm; AVAILABILITY: Unavailable; DESCRIPTION: Module: combo; GPIO, I2C x2, I2S x2, SDIO, SPI x3, UART x3; 19.5dBm; MF: Olimex LTD; MP: ESP-WROOM-32; PACKAGE: Module Espressif Systems; PRICE: None
U8 = SparkFun-IC-Conversion:VTI7064
U11 = ftdi:FT232R: Source: http://www.ftdichip.com/Documents/DataSheets/DS_FT232R_v104.pdf; MPN: FT232RL; OC_FARNELL: 1146032; OC_NEWARK: 91K9918
X1 X4 = micro usb B - 4LEGS:LCSC_MICRO_USB_4_LEGS
X3 = thumbpot:THUMBPOT
X6 X9 = SparkFun-Connectors:AUDIO_JACK_3.5MM: Audio Jack 3.5mm variants of PTH and SMT stereo audio jack with bypass switches. SparkFun Products: SparkFun SparkPunk Sound Kit - PTH MP3 Trigger -3.5mm SMD SparkFun PicoBoard- 2.5mm SMD; PROD_ID: CONN-08774; SF_ID: PRT-08032
X7 = PIC32MZ2048EFH144 Dev Board - FPC Final (5V LCD):SD-MMC_TF-HOLDER: TF / Micro SD socket is PUSH-PUSH type, the card can be pushed into and auto locked and pushed out by simply press the card. Surface Mounting type.
X8 = con-berg:PN87520: BERG USB connector; OC_FARNELL: unknown; OC_NEWARK: unknown
Y1 = SparkFun-Clocks:OSCILLATOR: Oscillators (Generic) These are active oscillators, which require a power source to generate their clock output. Most oscillators are configured to generate a set frequency (e.g. 16MHz). They have four pins: power, ground, output, and an enable input.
